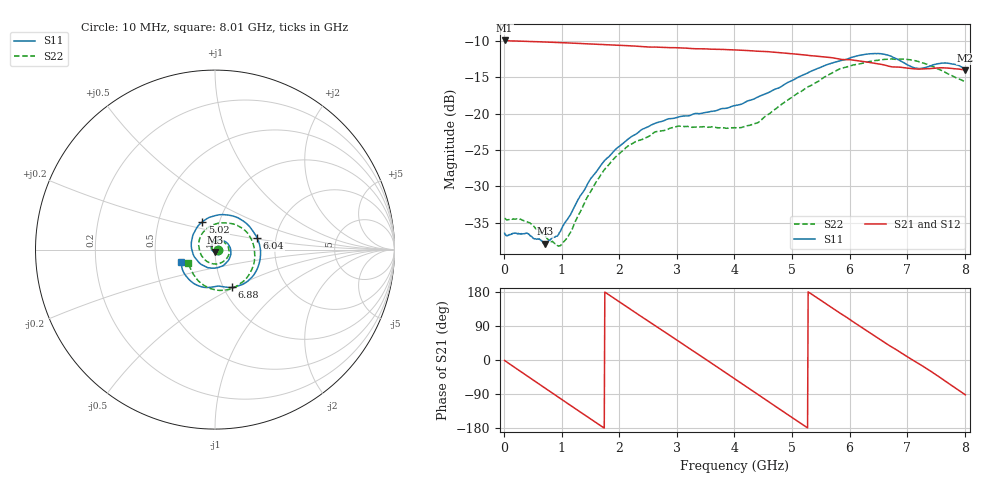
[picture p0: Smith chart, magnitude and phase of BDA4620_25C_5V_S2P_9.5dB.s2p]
!Agilent Technologies,E5071B,MY42404982,A.09.10
!Date: Wed May 06 09:00:08 2026
!Data & Calibration Information:
!Freq	S11:SOLT2(ON)	S21:SOLT2(ON)	S12:SOLT2(ON)	S22:SOLT2(ON)
# Hz S RI R 50
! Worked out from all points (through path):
!   801 points, 10 MHz to 8.01 GHz, reference 50 ohm
!   highest |S21| = -9.95 dB at 10 MHz (marker M1); lowest = -14.0 dB at 8.01 GHz (marker M2)
!   group delay of S21, straight-line fit = 281 ps
!   lowest |S11| = -37.9 dB at 710 MHz (marker M3), VSWR 1.03, Z = 49.9 - j1.27 ohm
!   |S11| at or under -10 dB: start of sweep to end of sweep
!   |S22| runs from -38.2 to -12.5 dB; largest |S21 - S12| = 0.0014
!   S11 on the Smith chart (normalised r, x): 10 MHz: 1.03, -0.00; 5.02 GHz: 0.83, +0.27; 6.04 GHz: 1.59, +0.22; 6.88 GHz: 1.10, -0.49; 8.01 GHz: 0.68, -0.10
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1e7  0.0151 -0.00103  0.318 -0.00678  0.3188 -0.00698  0.0191 -0.00119
3.3e8  0.0122 -0.00869  0.2582 -0.1784  0.2587 -0.1791  0.0162 -0.00885
7.1e8  -0.00124 -0.0127  0.0853 -0.2985  0.0851 -0.299  0.00293 -0.0141
9.8e8  -0.0144 -0.00592  -0.0634 -0.3009  -0.0635 -0.3013  -0.00946 -0.00804
1.35e9  -0.0213 0.0185  -0.2318 -0.195  -0.2321 -0.1951  -0.0174 0.0138
1.64e9  -0.00902 0.0409  -0.2943 -0.0542  -0.2946 -0.0542  -0.00911 0.0346
1.94e9  0.0185 0.054  -0.2772 0.1017  -0.2777 0.102  0.0139 0.0487
2.32e9  0.0608 0.0417  -0.1496 0.2486  -0.1502 0.2489  0.0505 0.0413
2.68e9  0.0874 0.000672  0.0254 0.2847  0.0256 0.2851  0.0744 0.0121
2.99e9  0.0812 -0.0473  0.1683 0.2282  0.1687 0.228  0.0776 -0.0249
3.39e9  0.0338 -0.0942  0.2719 0.0634  0.2725 0.063  0.0444 -0.0676
4.01e9  -0.0825 -0.078  0.1752 -0.2103  0.1754 -0.2108  -0.0508 -0.062
4.5e9  -0.1325 0.0262  -0.0482 -0.2632  -0.0486 -0.2638  -0.0907 0.0214
5.02e9  -0.0697 0.1553  -0.2309 -0.1141  -0.2314 -0.1139  -0.032 0.1275
5.35e9  0.031 0.1946  -0.2477 0.0315  -0.2479 0.0317  0.0524 0.1486
6.04e9  0.2348 0.0662  -0.0527 0.2279  -0.0529 0.2282  0.2113 0.0358
6.36e9  0.2485 -0.0683  0.0743 0.2115  0.0745 0.2117  0.2197 -0.0641
6.68e9  0.1695 -0.1853  0.1645 0.1331  0.165 0.1335  0.1754 -0.1593
6.88e9  0.0954 -0.2102  0.1953 0.0725  0.1959 0.0726  0.1253 -0.2006
7.19e9  0.0172 -0.203  0.1996 -0.0313  0.2005 -0.0311  0.0227 -0.2275
7.56e9  -0.0845 -0.2038  0.1459 -0.1458  0.1465 -0.1461  -0.0831 -0.1825
8.01e9  -0.1877 -0.0713  -0.0067 -0.1987  -0.00649 -0.1994  -0.1478 -0.072
